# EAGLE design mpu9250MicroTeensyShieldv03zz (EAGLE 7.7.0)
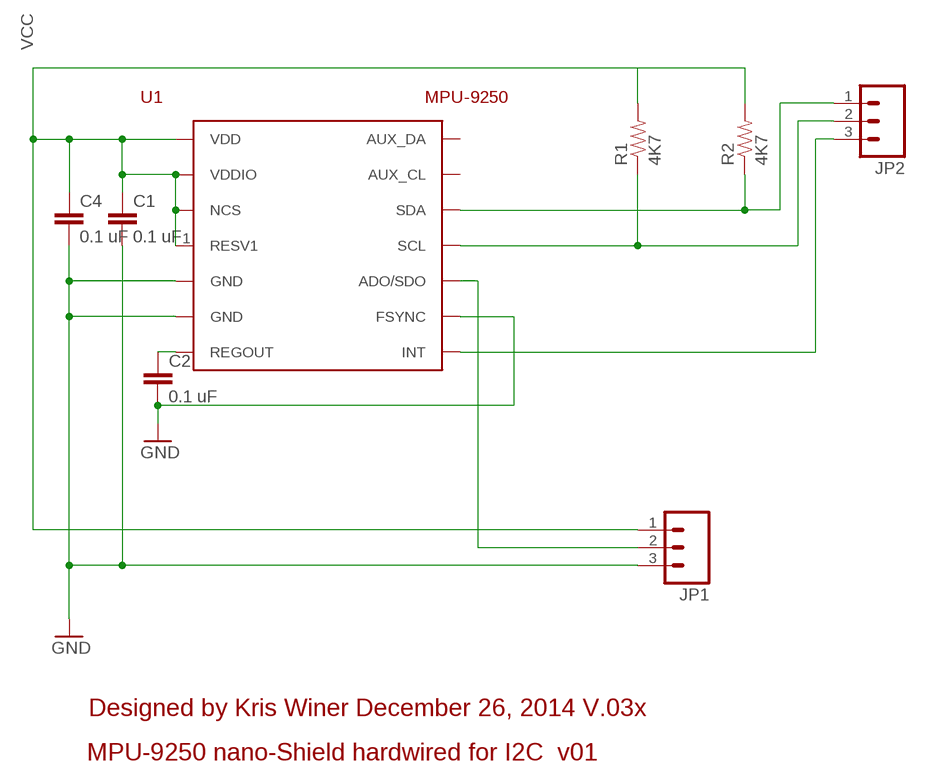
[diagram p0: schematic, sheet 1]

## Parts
C1  0.1 uF  0402CAP.KW  [0402-CAP]
C2  0.1 uF  0402CAP.KW  [0402-CAP]
C4  0.1 uF  0402CAP.KW  [0402-CAP]
JP1  M031X03_NO_SILK  [1X03_NO_SILK]
JP2  M031X03_NO_SILK  [1X03_NO_SILK]
R1  4K7  0402RES.KW  [0402-RES]
R2  4K7  0402RES.KW  [0402-RES]
U1  MPU-9250  [MPU-9250]

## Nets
GND: C1.2 C2.2 C4.2 JP1.3 U1.11(FSYNC) U1.18(GND) U1.20(GND)
N$1: JP2.1 R2.1 U1.24(SDA)
N$2: JP2.2 R1.1 U1.23(SCL)
N$3: C2.1 U1.10(REGOUT)
N$4: JP2.3 U1.12(INT)
N$7: JP1.2 U1.9(ADO/SDO)
VCC: C1.1 C4.1 JP1.1 R1.2 R2.2 U1.1(RESV1) U1.8(VDDIO) U1.13(VDD) U1.22(NCS)
Unconnected: U1.7(AUX_CL) U1.21(AUX_DA)

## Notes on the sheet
- Designed by Kris Winer December 26, 2014 V.03x
- MPU-9250 nano-Shield hardwired for I2C  v01

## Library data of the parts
C1 C2 C4 = SparkFun-Capacitors:0402CAP.KW
JP1 JP2 = SparkFun-Connectors:M03: Header 3 Standard 3-pin 0.1" header. Use with straight break away headers (SKU : PRT-00116), right angle break away headers (PRT-00553), swiss pins (PRT-00743), machine pins (PRT-00117), and female headers (PRT-00115). Molex polarized connector foot print use with SKU : PRT-08232 with associated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
R1 R2 = SparkFun-Resistors:0402RES.KW
U1 = SparkFun-Sensors:MPU-9250: The MPU-9250 is a 9-axis motion sensor that contains an accelerometer/gyro sensor (MPU-6500) combined with a magnetometer (AK8963).

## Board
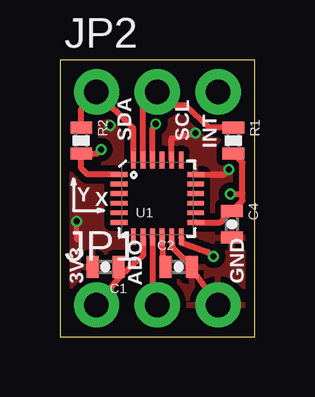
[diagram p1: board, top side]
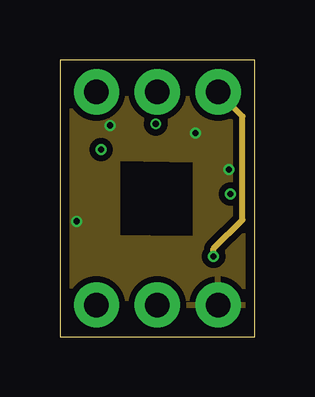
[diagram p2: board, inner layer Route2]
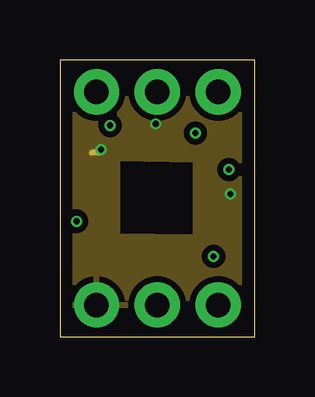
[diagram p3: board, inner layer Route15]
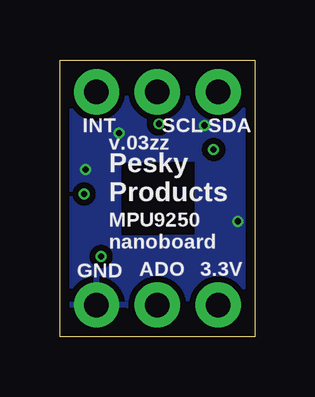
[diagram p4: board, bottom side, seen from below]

Size 8.13 x 11.56 mm. Coordinates in mm from the lower left corner, seen from the top.
Outline: 0,0 8.13,0 8.13,11.56 0,11.56 0,0
Copper layers (1*2*15*16): Top 0.035559375mm / dielectric 0.17018125mm / Route2 0.01778125mm / dielectric 47mil / Route15 0.01778125mm / dielectric 0.17018125mm / Bottom 0.035559375mm
Design rules "OSHPark-4layer *": minimum track width 5mil, minimum drill 10mil, track to track 5mil, track to pad 5mil, pad to pad 5mil, via to via 5mil, smd to smd 5mil, copper to edge 15mil, drill to drill 6mil, minimum pad ring 4mil, minimum via ring 4mil, stop-mask expansion 4mil, vias tented up to drill 20mil, thermal gap 10mil

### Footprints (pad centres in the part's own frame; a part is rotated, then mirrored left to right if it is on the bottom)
0402-CAP = smd 0.5 x 0.9: 1 -0.55,0; 2 0.55,0
1X03_NO_SILK = drill 1.016 pad 1.88: 1 0,0; 2 2.54,0; 3 5.08,0
0402-RES = smd 0.5 x 0.9: 1 -0.55,0; 2 0.55,0
MPU-9250 = smd 0.7 x 0.2: 1 -1.6,1; 2 -1.6,0.6; 3 -1.6,0.2; 4 -1.6,-0.2; 5 -1.6,-0.6; 6 -1.6,-1; 13 1.6,-1; 14 1.6,-0.6; 15 1.6,-0.2; 16 1.6,0.2; 17 1.6,0.6; 18 1.6,1 | smd 0.2 x 0.7: 7 -1,-1.6; 8 -0.6,-1.6; 9 -0.2,-1.6; 10 0.2,-1.6; 11 0.6,-1.6; 12 1,-1.6; 19 1,1.6; 20 0.6,1.6; 21 0.2,1.6; 22 -0.2,1.6; 23 -0.6,1.6; 24 -1,1.6

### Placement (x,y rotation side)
C1  1.91,2.92 180 top
C2  4.95,2.92 0 top
C4  7.18,4.7 270 top
JP1  1.52,1.33 0 top
JP2  1.52,10.22 0 top
R1  7.24,8.19 270 top
R2  0.89,8.19 270 top
U1  4.06,5.78 0 top

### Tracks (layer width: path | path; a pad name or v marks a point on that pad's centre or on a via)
GND  (via drill 0.25)
  Top 0.203: 6.87,6.78 v7.05,6.99 | 0.7,4.06 v0.7,4.83 | 5.52,2.9 C2.2
  Top 0.254: JP1.3 5.65,2.65 5.52,2.9 | U1.11 4.67,3.75 C2.2 | U1.20 4.66,8.28 v5.65,8.51 | U1.18 6.87,6.78
  Bottom 0.203: v5.65,8.51 5.65,8.64 | v7.05,6.99 7.11,6.99
  other vias: 2.1,8.83
  pour Route2 (isolate 0.254): 0,11.56 8.13,11.56 8.13,0 0,0 0,4.19 5.65,4.13 5.65,7.37 2.41,7.43 2.41,4.19 0,4.25
  pour Bottom (isolate 0.254): 0,11.56 8.13,11.56 8.13,0 0,0 0,4.19 5.65,4.13 5.65,7.37 2.41,7.43 2.41,4.19 0,4.25
  pour Top (isolate 0.254): 0,11.56 8.13,11.56 8.13,0 0,0 0,4.19 5.65,4.19 5.65,7.37 2.41,7.43 2.41,4.25 0,4.25
N$1
  Top 0.254: U1.24 3.06,8.68 JP2.1 0.89,9.52 R2.1
N$2
  Top 0.254: U1.23 3.46,9.62 JP2.2 4.64,9.65 5.27,9.65 6.25,8.74 R1.1
N$3
  Top 0.254: U1.10 4.27,3.31 C2.1
N$4  (via drill 0.25)
  Top 0.203: U1.12 5.06,4.14
  Top 0.254: 5.06,4.14 5.08,3.94 6.16,3.56 v6.41,3.37
  Route2 0.254: v6.41,3.37 6.41,3.68 7.62,4.89 7.62,9.21 JP2.3
N$7
  Top 0.203: 3.86,1.78 3.87,1.52 JP1.2
  Top 0.254: U1.9 3.86,1.78
VCC  (via drill 0.25)
  Top 0.203: 2.52,2.52 C1.1 2.62,2.64 | R2.2 1.17,7.64 | C4.1 7.18,5.4
  Top 0.254: U1.22 3.86,8.69 v4,8.89 | U1.13 6.69,4.78 C4.1 7.62,5.69 7.62,5.97 | U1.8 3.46,3.4 2.62,2.64 | 2.52,2.52 JP1.1 | 7.62,5.97 7.62,7.26 R1.2 | v7.11,5.97 7.62,5.97 | U1.1 1.16,6.78 0.89,7.05 R2.2 | 1.17,7.64 1.55,7.64 v1.71,7.81
  Route15 0.203: v4,8.89 3.87,8.83
  Route15 0.254: v7.11,5.97 7.18,5.97 | v1.71,7.81 1.65,7.68 1.33,7.68
  pour Route15 (isolate 0.254): 0.64,10.86 7.49,10.86 7.49,0.63 0.64,0.63 0.64,4.25 5.65,4.19 5.65,7.37 2.41,7.43 2.41,4.32 0.64,4.32

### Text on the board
tPlace: SDA | SCL | INT | Y | X | 3V3 | ADO | GND
bPlace: SDA | SCL | INT | v.03zz | Pesky / Products | MPU9250 / nanoboard | 3.3V | ADO | GND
